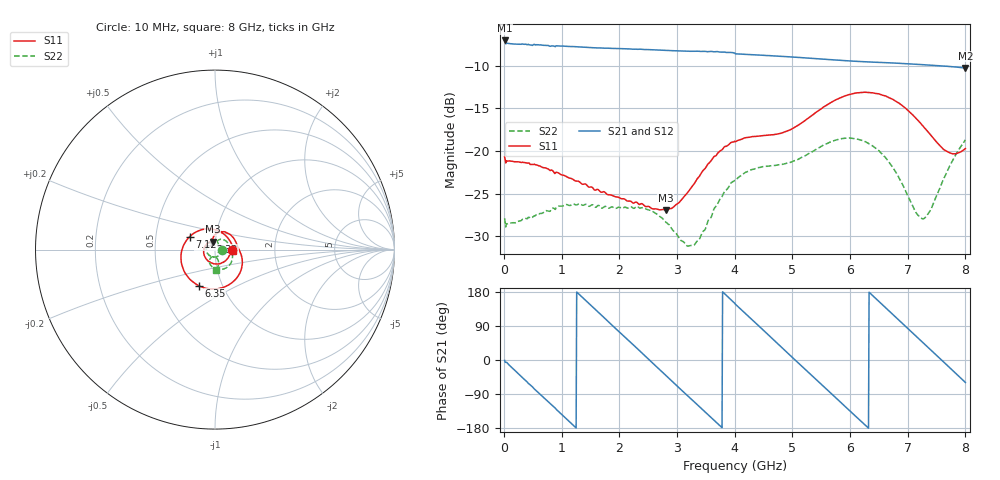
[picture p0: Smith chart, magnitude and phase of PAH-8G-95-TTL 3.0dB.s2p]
! MTS Systemtechnik GmbH
! S-Parameters
! Model: PAH-8G/95-TTL
! Attenuation Step: 3.0dB
! Rohde & Schwarz ZVB8 2Ports - Version 4.11 - 1145.1010k08 SN: 100119
! S2P File Measurements:
! S11 S21 S12 S22
# HZ  S  DB  R  50.00
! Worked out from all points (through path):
!   800 points, 10 MHz to 8 GHz, reference 50 ohm
!   highest |S21| = -7.01 dB at 10 MHz (marker M1); lowest = -10.2 dB at 8 GHz (marker M2)
!   group delay of S21, straight-line fit = 395 ps
!   lowest |S11| = -26.9 dB at 2.8 GHz (marker M3), VSWR 1.09, Z = 48.7 + j4.25 ohm
!   |S11| at or under -10 dB: start of sweep to end of sweep
!   |S22| runs from -31.2 to -18.5 dB; largest |S21 - S12| = 0.0057
!   S11 on the Smith chart (normalised r, x): 10 MHz: 1.20, -0.01; 2.32 GHz: 0.95, +0.08; 6.35 GHz: 0.77, -0.33; 7.12 GHz: 0.75, +0.11; 8 GHz: 1.23, -0.03
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1e7  -20.71 -3.0  -7.01 -1.1  -6.93 -1.0  -27.91 -6.3
3.8e8  -21.38 -49.3  -7.45 -55.2  -7.46 -55.2  -27.93 -66.3
6.5e8  -21.88 -83.8  -7.56 -93.9  -7.55 -93.9  -27.34 -110.3
1.03e9  -22.85 -131.4  -7.67 -148.0  -7.68 -148.0  -26.43 -163.3
1.35e9  -23.88 -168.2  -7.79 166.5  -7.79 166.5  -26.34 159.8
1.84e9  -25.15 147.3  -7.93 96.6  -7.94 96.7  -26.65 118.8
2.32e9  -26.15 116.3  -8.05 28.9  -8.04 28.9  -26.53 88.6
2.68e9  -26.89 105.4  -8.14 -22.8  -8.14 -22.6  -27.57 66.9
2.8e9  -26.92 104.8  -8.18 -39.8  -8.17 -39.8  -28.32 61.1
3.32e9  -23.60 99.6  -8.28 -113.5  -8.30 -113.9  -30.86 70.7
3.69e9  -20.41 80.4  -8.31 -165.6  -8.33 -165.6  -26.38 75.3
4.01e9  -18.92 55.8  -8.57 147.5  -8.57 147.4  -23.49 56.7
4.56e9  -18.16 20.1  -8.78 69.4  -8.80 69.4  -21.80 22.2
4.96e9  -17.52 0.8  -8.94 12.4  -8.94 12.3  -21.35 3.4
5.34e9  -15.82 -20.4  -9.11 -41.4  -9.12 -41.4  -20.10 -13.8
5.8e9  -13.84 -57.6  -9.32 -106.3  -9.34 -106.5  -18.63 -43.5
6.35e9  -13.13 -114.1  -9.54 175.9  -9.55 175.9  -19.23 -86.2
6.67e9  -13.72 -150.4  -9.63 130.6  -9.64 130.7  -21.27 -108.2
7.12e9  -15.99 153.2  -9.80 66.5  -9.80 66.5  -26.95 -112.4
7.3e9  -17.35 126.9  -9.87 40.8  -9.87 40.8  -27.84 -92.4
7.56e9  -19.36 83.0  -9.98 3.8  -9.98 3.7  -24.32 -73.9
8e9  -19.71 -5.7  -10.24 -59.2  -10.24 -59.2  -18.68 -87.6
